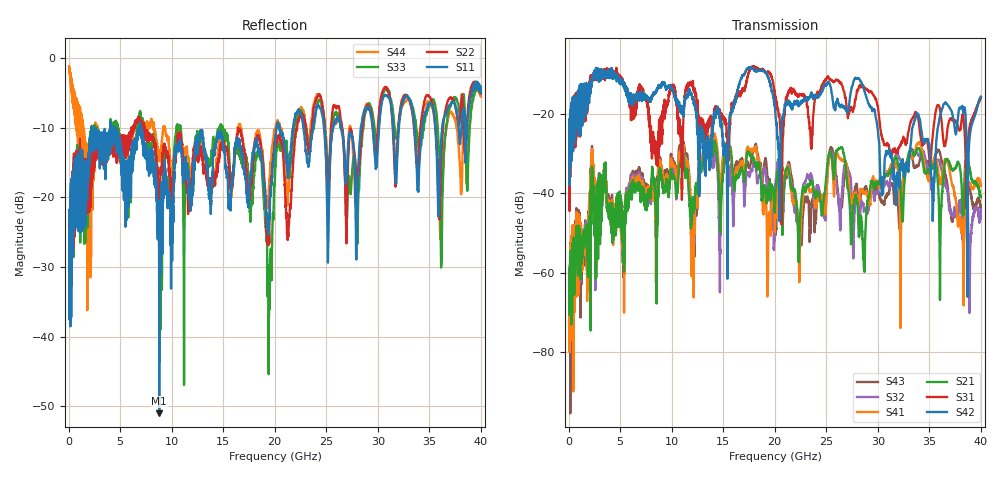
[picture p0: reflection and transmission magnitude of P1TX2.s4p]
!Agilent Technologies,N5245A,MY49151084,A.09.20.08
!Agilent N5245A: A.09.20.08
!Date: Thursday, March 01, 2012 13:20:12
!Correction: S11(Full 4 Port(1,2,3,4))
!S12(Full 4 Port(1,2,3,4))
!S13(Full 4 Port(1,2,3,4))
!S14(Full 4 Port(1,2,3,4))
!S21(Full 4 Port(1,2,3,4))
!S22(Full 4 Port(1,2,3,4))
!S23(Full 4 Port(1,2,3,4))
!S24(Full 4 Port(1,2,3,4))
!S31(Full 4 Port(1,2,3,4))
!S32(Full 4 Port(1,2,3,4))
!S33(Full 4 Port(1,2,3,4))
!S34(Full 4 Port(1,2,3,4))
!S41(Full 4 Port(1,2,3,4))
!S42(Full 4 Port(1,2,3,4))
!S43(Full 4 Port(1,2,3,4))
!S44(Full 4 Port(1,2,3,4))
!S4P File: Measurements: <S11,S12,S13,S14>,
!<S21,S22,S23,S24>,
!<S31,S32,S33,S34>,
!<S41,S42,S43,S44>:
# Hz S  dB  R 50
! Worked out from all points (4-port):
!   3996 points, 50 MHz to 40 GHz, reference 50 ohm
!   strongest paths, dB at 50 MHz, 10.04 GHz, 20.03 GHz, 30.02 GHz, 40 GHz:
!     S42: -24.8, -13.7, -18.9, -24.6, -15.7
!     S31: -25.6, -13.1, -15.2, -18.5, -16.0
!     S21: -65.7, -36.0, -42.6, -37.9, -41.1
!     S41: -73.8, -32.9, -46.8, -37.8, -38.2
!     S32: -69.7, -34.9, -40.8, -39.5, -44.1
!     S43: -67.5, -31.9, -50.4, -39.2, -43.4
!   lowest |S11| = -51.0 dB at 8.79 GHz (marker M1), VSWR 1.01, Z = 49.7 - j0.11 ohm
!   |S11| at or under -10 dB: start of sweep to 2.235 GHz; 4.411 GHz to 6.858 GHz (2.447 GHz wide, 43.4 % of centre); 7.003 GHz to 20.18 GHz (13.17 GHz wide, 96.9 % of centre)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
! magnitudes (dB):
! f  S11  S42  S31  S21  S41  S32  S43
! 50 MHz  -23.9  -24.8  -25.6  -65.7  -73.8  -69.7  -67.5
! 2.34 GHz  -13.5  -10.8  -11.6  -35.9  -30.8  -36.3  -30.6
! 8.79 GHz  -51.0  -13.1  -22.4  -34.9  -32.5  -32.8  -30.8
! 15.28 GHz  -15.9  -30.2  -22.7  -29.0  -27.7  -29.0  -32.1
! 28.02 GHz  -20.1  -11.0  -14.3  -42.5  -40.8  -41.6  -39.6
! 35.32 GHz  -7.0  -46.6  -25.7  -33.8  -32.2  -39.8  -32.8
! 40 GHz  -5.0  -15.7  -16.0  -41.1  -38.2  -44.1  -43.4
